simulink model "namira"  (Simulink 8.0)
settings: Solver=ode45  StartTime=0.0  StopTime=0.021  MaxStep=0.1e-6  RelTol=1e-3
InitFcn:
  | clc;
  | clear;
  | L = 4.1e-6;
  | RL = 80e-3;
  | C = 376e-6;
  | Rc = 5e-3;
  | fs = 100e3;
  | Vg = 12;
  | D = 0.42;
  | R = 1;
StopFcn:
  | clc;
libraries: powerlib x9, fl_lib x3, nesl_utility x2, simulink x1, elec_lib x1

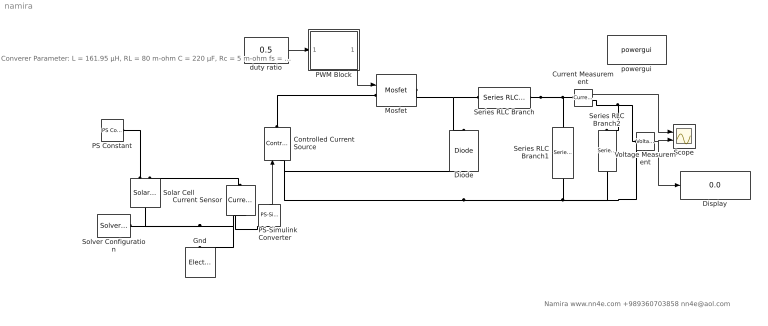
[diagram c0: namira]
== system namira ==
  note: Namira www.nn4e.com +989360703858 nn4e@aol.com
  note: Converer Parameter: L = 161.95 µH, RL = 80 m-ohm C = 220 µF, Rc = 5 m-ohm fs = 100 KHz, Vg = 24 D = 0.53, Load R = 10 ohm
  Controlled Current Source : powerlib/Electrical Sources/Controlled Current Source  Initialize=on  Source_Type=AC  Amplitude=0  Phase=0  Frequency=0  Measurements=None
  Current Measurement : powerlib/Measurements/Current Measurement  PhasorSimulation=off  OutputType=Complex  PSBequivalent=0
  Current Sensor : fl_lib/Electrical/Electrical Sensors/Current Sensor  i1_Log=off  v1_Log=off  LocalVarNames=|i1|v1  LocalVarDescs=|i1|v1  LocalVarLogging=[0 0]
  Diode : powerlib/Power Electronics/Diode  Ron=0.001  Lon=0  Vf=0.8  IC=0  UseSnubber=off  Rs=500  Cs=250e-9  Measurements=off
  Display : Display
  Gnd : fl_lib/Electrical/Electrical Elements/Electrical Reference  i_Log=off  LocalVarNames=|i  LocalVarDescs=|i  LocalVarLogging=[]
  Mosfet : powerlib/Power Electronics/Mosfet  Ron=0.1  Lon=0  Rd=0.01  Vfd=0  IC=0  Rs=1e5  Cs=inf  Measurements=off
  PS Constant : fl_lib/Physical Signals/Sources/PS Constant  constant=500  LocalVarLogging=[]
  PS-Simulink Converter : nesl_utility/PS-Simulink Converter  PhysicalDomain=network_engine_domain  LeftPortType=input  RightPortType=output  SubClassName=ps_output  PseudoPeriodic=off  Frequencies=[]  Unit=1  AffineConversion=off
  PWM Block : Subsystem
  Scope : Scope  NumInputPorts=2
  Series RLC Branch : powerlib/Elements/Series RLC Branch  LConnTagsString=__new0  RConnTagsString=__new0  BranchType=RL  Resistance=RL  Inductance=161.95e-6  SetiL0=off  InitialCurrent=0  Capacitance=1e-6  Setx0=off  InitialVoltage=0  Measurements=None
  Series RLC Branch1 : powerlib/Elements/Series RLC Branch  LConnTagsString=__new0  RConnTagsString=__new0  BranchType=RC  Resistance=Rc  Inductance=1e-3  SetiL0=off  InitialCurrent=0  Capacitance=220e-6  Setx0=off  InitialVoltage=0  Measurements=None
  Series RLC Branch2 : powerlib/Elements/Series RLC Branch  LConnTagsString=__new0  RConnTagsString=__new0  BranchType=R  Resistance=10  Inductance=1e-3  SetiL0=off  InitialCurrent=0  Capacitance=1e-6  Setx0=off  InitialVoltage=0  Measurements=Branch voltage and current
  Solar Cell : elec_lib/Sources/Solar Cell  prm=1  Isc=7.34 A  Voc=0.6 V  Is=1e-6 A  Is2=0 A  Iph=7.34 A  Ir0=1000 W/m^2  ec=1.5  N2=2  Rs=0 Ohm  Rp=Inf Ohm  TIPH1=0 1/K  EG=1.11 eV  TXIS1=3  TXIS2=3  TRS1=0  TRP1=0  Tmeas=25 C  TFIXED=25 C  LocalVarLogging=[]  thermal_mass=100 J/K  initial_temperature=25 C
  Solver Configuration : nesl_utility/Solver Configuration  PhysicalDomain=network_engine_domain  LeftPortType=input  RightPortType=generic  SubClassName=solver  Accelerate=off  Profile=off  UseLocalSampling=off  FrequencyDomain=off  Tones=[]  Harmonics=[]  UseCCode=off  SimulateNoise=off  EnableSwitchedLinearOptims=on  DoDC=off  ResidualTolerance=1e-9  UseLocalSolver=off  LocalSolverChoice=NE_TRAPEZOIDAL_ADVANCER  LocalSolverSampleTime=.001  DoFixedCost=off  MaxNonlinIter=3  MaxModeIter=2  LinearAlgebra=Sparse  DelaysMemoryBudget=1024
  Voltage Measurement : powerlib/Measurements/Voltage Measurement  PhasorSimulation=off  OutputType=Complex  PSBequivalent=0
  duty ratio : Constant  Value=0.5
  powergui : powerlib/powergui  Priority=1  SimulationMode=Continuous  SolverType=Tustin  SampleTime=1e-8  frequency=60  SPID=off  DisableSnubberDevices=off  DisableRonSwitches=off  DisableVfSwitches=off  SwTol=0  Interpol=off  DisplayEquations=off  FunctionMessages=off  frequencyindice=0  Pbase=100e6  ErrMax=1e-4  Iterations=50  UnitsV=kV  UnitsW=MW  echomessages=off  HookPort=off  EnableUseOfTLC=off  x0status=blocks  RestoreLinks=warning  ResistiveCurrentMeasurement=off  Frange=[0:2:500]  Ylog=off  Xlog=on  ShowGrid=off  save=off  variable=ZData  structure=tpa14cfcc1_35b5_40eb_8b70_049b43167a68  ZoomFFT=off  StartTime=0.0  cycles=1  DisplayStyle=1  fundamental=60  FreqAxis=off  MaxFrequency=1000  frequencyindicesteady=1  RmsSteady=1  display=off  Ts=0  methode=off
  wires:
  duty ratio/1 -> PWM Block/1(d)
  Current Measurement/1 -> Scope/1
  PWM Block/1(c) -> Mosfet/1
  Voltage Measurement/1 -> Scope/2, Display/1
  PS-Simulink Converter/1 -> Controlled Current Source/1
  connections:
  Controlled Current Source/RConn1 -- Mosfet/LConn1
  Mosfet/RConn1 -- Diode/RConn1 -- Series RLC Branch/LConn1
  Controlled Current Source/LConn1 -- Voltage Measurement/LConn2 -- Series RLC Branch2/RConn1 -- Series RLC Branch1/RConn1 -- Diode/LConn1
  Voltage Measurement/LConn1 -- Series RLC Branch2/LConn1 -- Current Measurement/RConn1
  Series RLC Branch/RConn1 -- Series RLC Branch1/LConn1 -- Current Measurement/LConn1
  Solar Cell/LConn1 -- PS Constant/RConn1
  Current Sensor/RConn1 -- PS-Simulink Converter/LConn1
  Solar Cell/LConn2 -- Current Sensor/LConn1
  Current Sensor/RConn2 -- Solar Cell/RConn1 -- Solver Configuration/RConn1 -- Gnd/LConn1

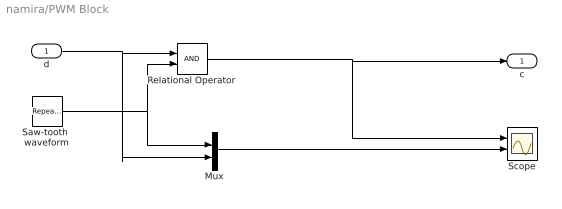
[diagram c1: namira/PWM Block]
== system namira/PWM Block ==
  d : Inport
  Mux : Mux  Inputs=2
  Relational Operator : RelationalOperator  OutDataTypeStr=boolean
  Saw-tooth  waveform : simulink/Sources/Repeating Sequence  rep_seq_t=[0 1/fs]  rep_seq_y=[0 1]
  Scope : Scope  NumInputPorts=2
  c : Outport
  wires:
  d/1 -> Mux/2, Relational Operator/1
  Saw-tooth  waveform/1 -> Mux/1, Relational Operator/2
  Relational Operator/1 -> c/1, Scope/1
  Mux/1 -> Scope/2
